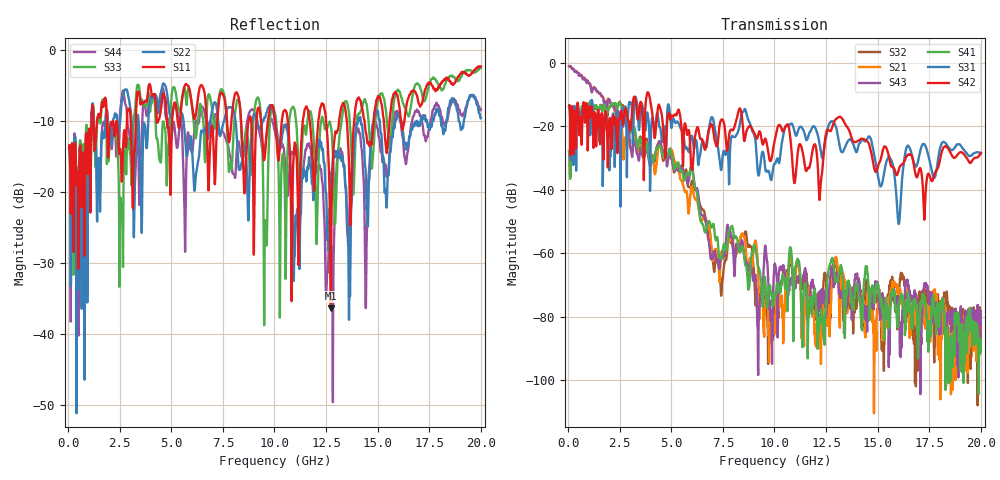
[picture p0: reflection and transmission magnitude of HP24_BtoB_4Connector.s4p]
# MHz S MA R 50.00
! FREQ  S11  S12  S13  S14
!  S21  S22  S23  S24
!  S31  S32  S33  S34
!  S41  S42  S43  S44
!  MAG  ANG  MAG  ANG  MAG  ANG  MAG  ANG
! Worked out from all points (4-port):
!   1996 points, 50 MHz to 20 GHz, reference 50 ohm
!   strongest paths, dB at 50 MHz, 5.04 GHz, 10.03 GHz, 15.02 GHz, 20 GHz:
!     S42: -13.7, -16.8, -23.9, -32.5, -28.4
!     S31: -13.7, -19.1, -31.8, -36.0, -28.6
!     S41: -27.9, -29.5, -73.9, -70.4, -91.1
!     S43: -1.1, -30.9, -63.6, -71.3, -81.8
!     S21: -1.1, -27.8, -81.2, -75.5, -84.0
!     S32: -27.8, -30.3, -76.1, -77.0, -83.0
!   lowest |S11| = -36.4 dB at 12.73 GHz (marker M1), VSWR 1.03, Z = 48.6 + j0.514 ohm
!   |S11| at or under -10 dB: start of sweep to 1.141 GHz; 10.64 GHz to 11.37 GHz (732.2 MHz wide, 6.65 % of centre); 12.5 GHz to 13.13 GHz (631.7 MHz wide, 4.93 % of centre)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
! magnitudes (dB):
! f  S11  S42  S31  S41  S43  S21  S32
! 50 MHz  -13.8  -13.7  -13.7  -27.9  -1.1  -1.1  -27.8
! 2.57 GHz  -16.2  -15.2  -20.0  -13.8  -18.0  -19.4  -13.4
! 9.22 GHz  -8.2  -22.5  -35.5  -64.4  -90.8  -68.2  -72.0
! 9.56 GHz  -14.1  -24.0  -33.7  -68.8  -57.8  -74.9  -77.0
! 12.73 GHz  -36.4  -21.5  -18.5  -63.0  -65.8  -75.9  -76.7
! 16.02 GHz  -7.5  -33.7  -50.8  -77.5  -79.7  -71.1  -75.8
! 20 GHz  -2.4  -28.4  -28.6  -91.1  -81.8  -84.0  -83.0
